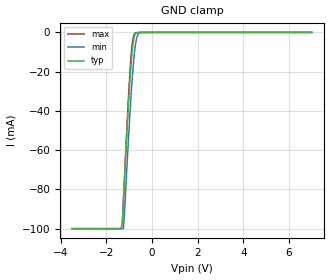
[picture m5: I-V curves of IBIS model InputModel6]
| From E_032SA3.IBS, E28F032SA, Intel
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|*************************Input Model 6****************************
[Model]   InputModel6
Model_type   Input
|   For CE#6
Vinl = 0.8V
Vinh = 2.0V
| Variable   typ   min   max
C_comp   5.61p   NA   7.6p
[Voltage Range]   3.3V   3.0V   3.6V
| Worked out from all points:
|   GND clamp passes 1 mA (typ) near -0.74 V on its own axis
[GND_clamp]
|Voltage I(typ)   I(min)   I(max)
-3.5V     -100mA     -100mA     -100mA
-1.35V    -100mA     -100mA     -100mA
-1.3V     -96.86mA   -100mA     -97.87mA
-1.25V    -84.98mA   -100mA     -84.88mA
-1.2V     -73.41mA   -91.03mA   -72.33mA
-1.1V     -51.11mA   -68.92mA   -48.19mA
-950mV    -21.39mA   -38.22mA   -17.02mA
-850mV    -7.392mA   -21.06mA   -4.215mA
-750mV    -1.193mA   -8.302mA   -476.6uA
-650mV    -170.6uA   -2.019mA   -100.8uA
-500mV    -14.35uA   -106.3uA   -6.47uA
7V        0A         0A         0A
[POWER_clamp]
| Input buffer circuits of this product do not intrinsically
| require a [POWER_clamp] definition.  This zero current
| [POWER_clamp] is provided for compatibility with some ibis
| parsers.
|   Voltage  I(typ)   I(min)   I(max)
-5V       0A         0A         0A
-4.75V    0A         0A         0A
9.75V     0A         0A         0A
10V       0A         0A         0A
